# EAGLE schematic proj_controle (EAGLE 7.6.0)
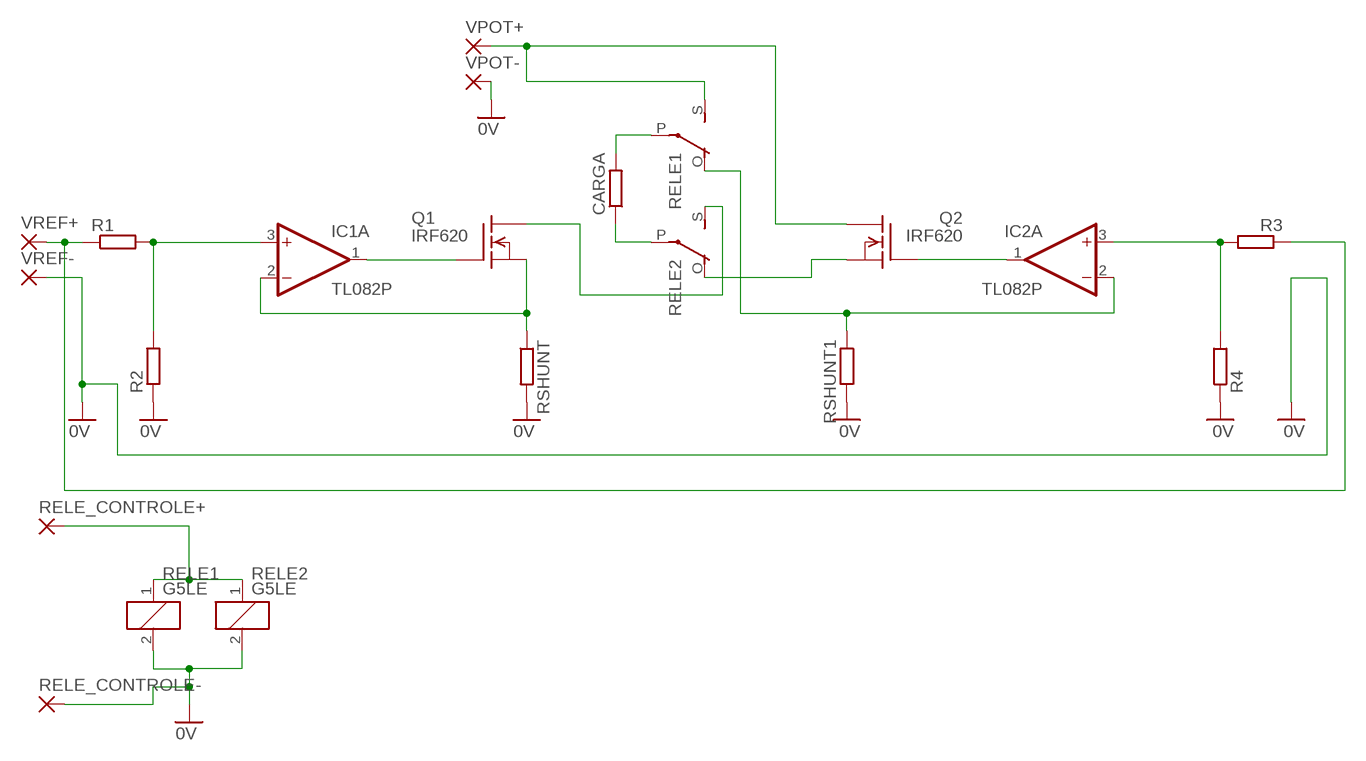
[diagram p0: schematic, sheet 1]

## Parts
CARGA  R-EU_0207/10  [0207/10]
IC1  TL082P  [DIL08]
IC2  TL082P  [DIL08]
Q1  IRF620  [TO220]
Q2  IRF620  [TO220]
R1  R-EU_0207/10  [0207/10]
R2  R-EU_0207/10  [0207/10]
R3  R-EU_0207/10  [0207/10]
R4  R-EU_0207/10  [0207/10]
RELE1  G5LE  [G5LE]
RELE2  G5LE  [G5LE]
RELE_CONTROLE+  3,17/1,1  [3,17/1,1]
RELE_CONTROLE-  3,17/1,1  [3,17/1,1]
RSHUNT  R-EU_0617/22  [0617/22]
RSHUNT1  R-EU_0617/22  [0617/22]
VPOT+  3,17/1,1  [3,17/1,1]
VPOT-  3,17/1,1  [3,17/1,1]
VREF+  3,17/1,1  [3,17/1,1]
VREF-  3,17/1,1  [3,17/1,1]

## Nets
0V: R2.1 R4.1 RELE1.2 RELE2.2 RELE_CONTROLE-.1(P) RSHUNT1.2 RSHUNT.2 VPOT-.1(P) VREF-.1(P)
N$1: CARGA.1 RELE2.P(2:P)
N$2: IC1.3(A:+IN) R1.2 R2.2
N$3: IC1.1(A:OUT) Q1.1(G)
N$4: IC1.2(A:-IN) Q1.3(S) RSHUNT.1
N$7: CARGA.2 RELE1.P(2:P)
N$8: Q1.2(D) RELE2.S(2:S)
N$9: IC2.3(A:+IN) R3.2 R4.2
N$10: IC2.1(A:OUT) Q2.1(G)
N$11: IC2.2(A:-IN) RELE1.O(2:O) RSHUNT1.1
N$12: R1.1 R3.1 VREF+.1(P)
N$13: Q2.2(D) RELE1.S(2:S) VPOT+.1(P)
N$14: Q2.3(S) RELE2.O(2:O)
N$15: RELE1.1 RELE2.1 RELE_CONTROLE+.1(P)
Unconnected: IC1.5(B:+IN) IC1.6(B:-IN) IC1.7(B:OUT) IC2.5(B:+IN) IC2.6(B:-IN) IC2.7(B:OUT)

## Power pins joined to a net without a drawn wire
V+: IC1.8(P:V+) IC2.8(P:V+)
V-: IC1.4(P:V-) IC2.4(P:V-)

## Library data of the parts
CARGA R1-R4 = rcl:R-EU_: RESISTOR, European symbol
IC1 IC2 = linear:TL082: OP AMP Data sheet; DATA_SHEET: <a href="http://www.ti.com/lit/ds/symlink/tl084a.pdf"> Data sheet </a>
Q1 Q2 = transistor-fet:IRF620: N-Channel Enhancement MOSFET (HEXFET); 200V; 5,2A; 0,8Ohm
RELE1 RELE2 = relay:G5LE: RELAY 1 x switch, 10 A/120 V AC, 8 A/30 V DC, Omron; OC_FARNELL: unknown; OC_NEWARK: unknown
RELE_CONTROLE+ RELE_CONTROLE- VPOT+ VPOT- VREF+ VREF- = wirepad:3,17/1,1: THROUGH-HOLE PAD
RSHUNT RSHUNT1 = resistor:R-EU_: RESISTOR, European symbol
